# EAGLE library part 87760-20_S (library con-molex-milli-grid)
HEADER
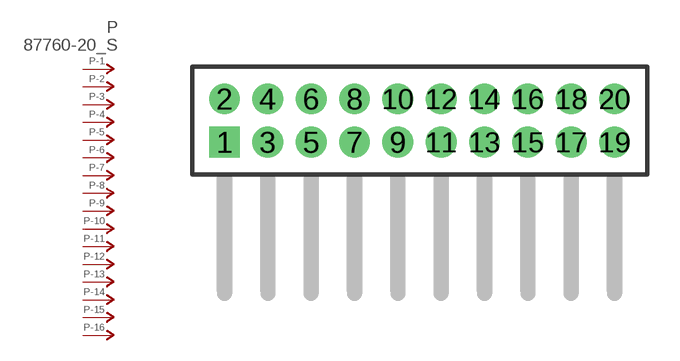
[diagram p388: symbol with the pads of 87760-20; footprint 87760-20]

Designator prefix P; gates -1=P-NV -2=P-N -3=P-N -4=P-N -5=P-N -6=P-N -7=P-N -8=P-N -9=P-N -10=P-N -11=P-N -12=P-N -13=P-N -14=P-N -15=P-N -16=P-N -17=P-N -18=P-N -19=P-N -20=P-N

## 87760-20_S  [87760-20]
1  -1:P  pas
2  -2:P  pas
3  -3:P  pas
4  -4:P  pas
5  -5:P  pas
6  -6:P  pas
7  -7:P  pas
8  -8:P  pas
9  -9:P  pas
10  -10:P  pas
11  -11:P  pas
12  -12:P  pas
13  -13:P  pas
14  -14:P  pas
15  -15:P  pas
16  -16:P  pas
17  -17:P  pas
18  -18:P  pas
19  -19:P  pas
20  -20:P  pas

## Footprint 87760-20 (pad centres in mm)
HEADER Dual Row, Right Angle
drill 0.914 square: 1 -9,-1
drill 0.914: 2 -9,1; 3 -7,-1; 4 -7,1; 5 -5,-1; 6 -5,1; 7 -3,-1; 8 -3,1; 9 -1,-1; 10 -1,1; 11 1,-1; 12 1,1; 13 3,-1; 14 3,1; 15 5,-1; 16 5,1; 17 7,-1; 18 7,1; 19 9,-1; 20 9,1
